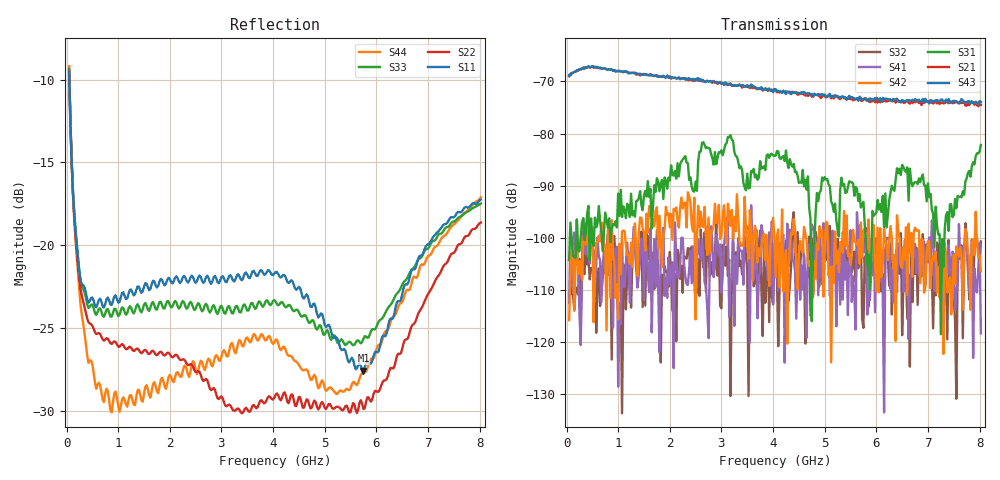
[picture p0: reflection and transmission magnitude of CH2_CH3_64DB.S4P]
!Agilent Technologies,E5071C,MY46316741,A.11.02
!Date: Thu May 28 14:42:12 2026
!Data & Calibration Information:
!1:CH2 INPUT 2:CH2 OUTPUT 3:CH3 INPUT 4:CH3 OUTPUT
!Freq	S11:SOLT4(ON)	S12:SOLT4(ON)	S13:SOLT4(ON)	S14:SOLT4(ON)
!	S21:SOLT4(ON)	S22:SOLT4(ON)	S23:SOLT4(ON)	S24:SOLT4(ON)
!	S31:SOLT4(ON)	S32:SOLT4(ON)	S33:SOLT4(ON)	S34:SOLT4(ON)
!	S41:SOLT4(ON)	S42:SOLT4(ON)	S43:SOLT4(ON)	S44:SOLT4(ON)
!PortZ  Port1:50+j0  Port2:50+j0  Port3:50+j0  Port4:50+j0
!Above PortZ is port z conversion or system Z0 setting when saving the data.
!When reading, reference impedance value at option line is always used.
# Hz S dB R 50
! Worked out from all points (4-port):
!   320 points, 50 MHz to 8.025 GHz, reference 50 ohm
!   strongest paths, dB at 50 MHz, 2.05 GHz, 4.05 GHz, 6.05 GHz, 8.025 GHz:
!     S43: -68.8, -69.2, -71.5, -73.5, -73.9
!     S21: -69.0, -69.3, -71.6, -73.4, -74.5
!     S31: -104.1, -87.9, -84.2, -94.6, -82.2
!     S42: -115.8, -100.4, -107.5, -110.4, -106.4
!     S41: -112.5, -104.7, -102.3, -103.4, -118.3
!     S32: -104.2, -113.9, -107.3, -104.1, -100.7
!   lowest |S11| = -27.6 dB at 5.75 GHz (marker M1), VSWR 1.09, Z = 47.1 - j2.87 ohm
!   |S11| at or under -10 dB: 53.76 MHz to end of sweep
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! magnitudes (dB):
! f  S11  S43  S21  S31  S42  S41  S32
! 50 MHz  -9.5  -68.8  -69.0  -104.1  -115.8  -112.5  -104.2
! 125 MHz  -16.9  -68.4  -68.4  -103.4  -102.5  -109.5  -111.1
! 275 MHz  -22.2  -67.6  -67.7  -99.7  -104.4  -120.5  -115.6
! 875 MHz  -23.6  -67.7  -67.8  -98.2  -96.6  -110.3  -123.3
! 4.075 GHz  -21.6  -71.9  -72.1  -83.3  -99.6  -106.0  -107.2
! 5.75 GHz  -27.6  -73.5  -73.4  -93.1  -98.7  -102.8  -117.2
! 8.025 GHz  -17.2  -73.9  -74.5  -82.2  -106.4  -118.3  -100.7
